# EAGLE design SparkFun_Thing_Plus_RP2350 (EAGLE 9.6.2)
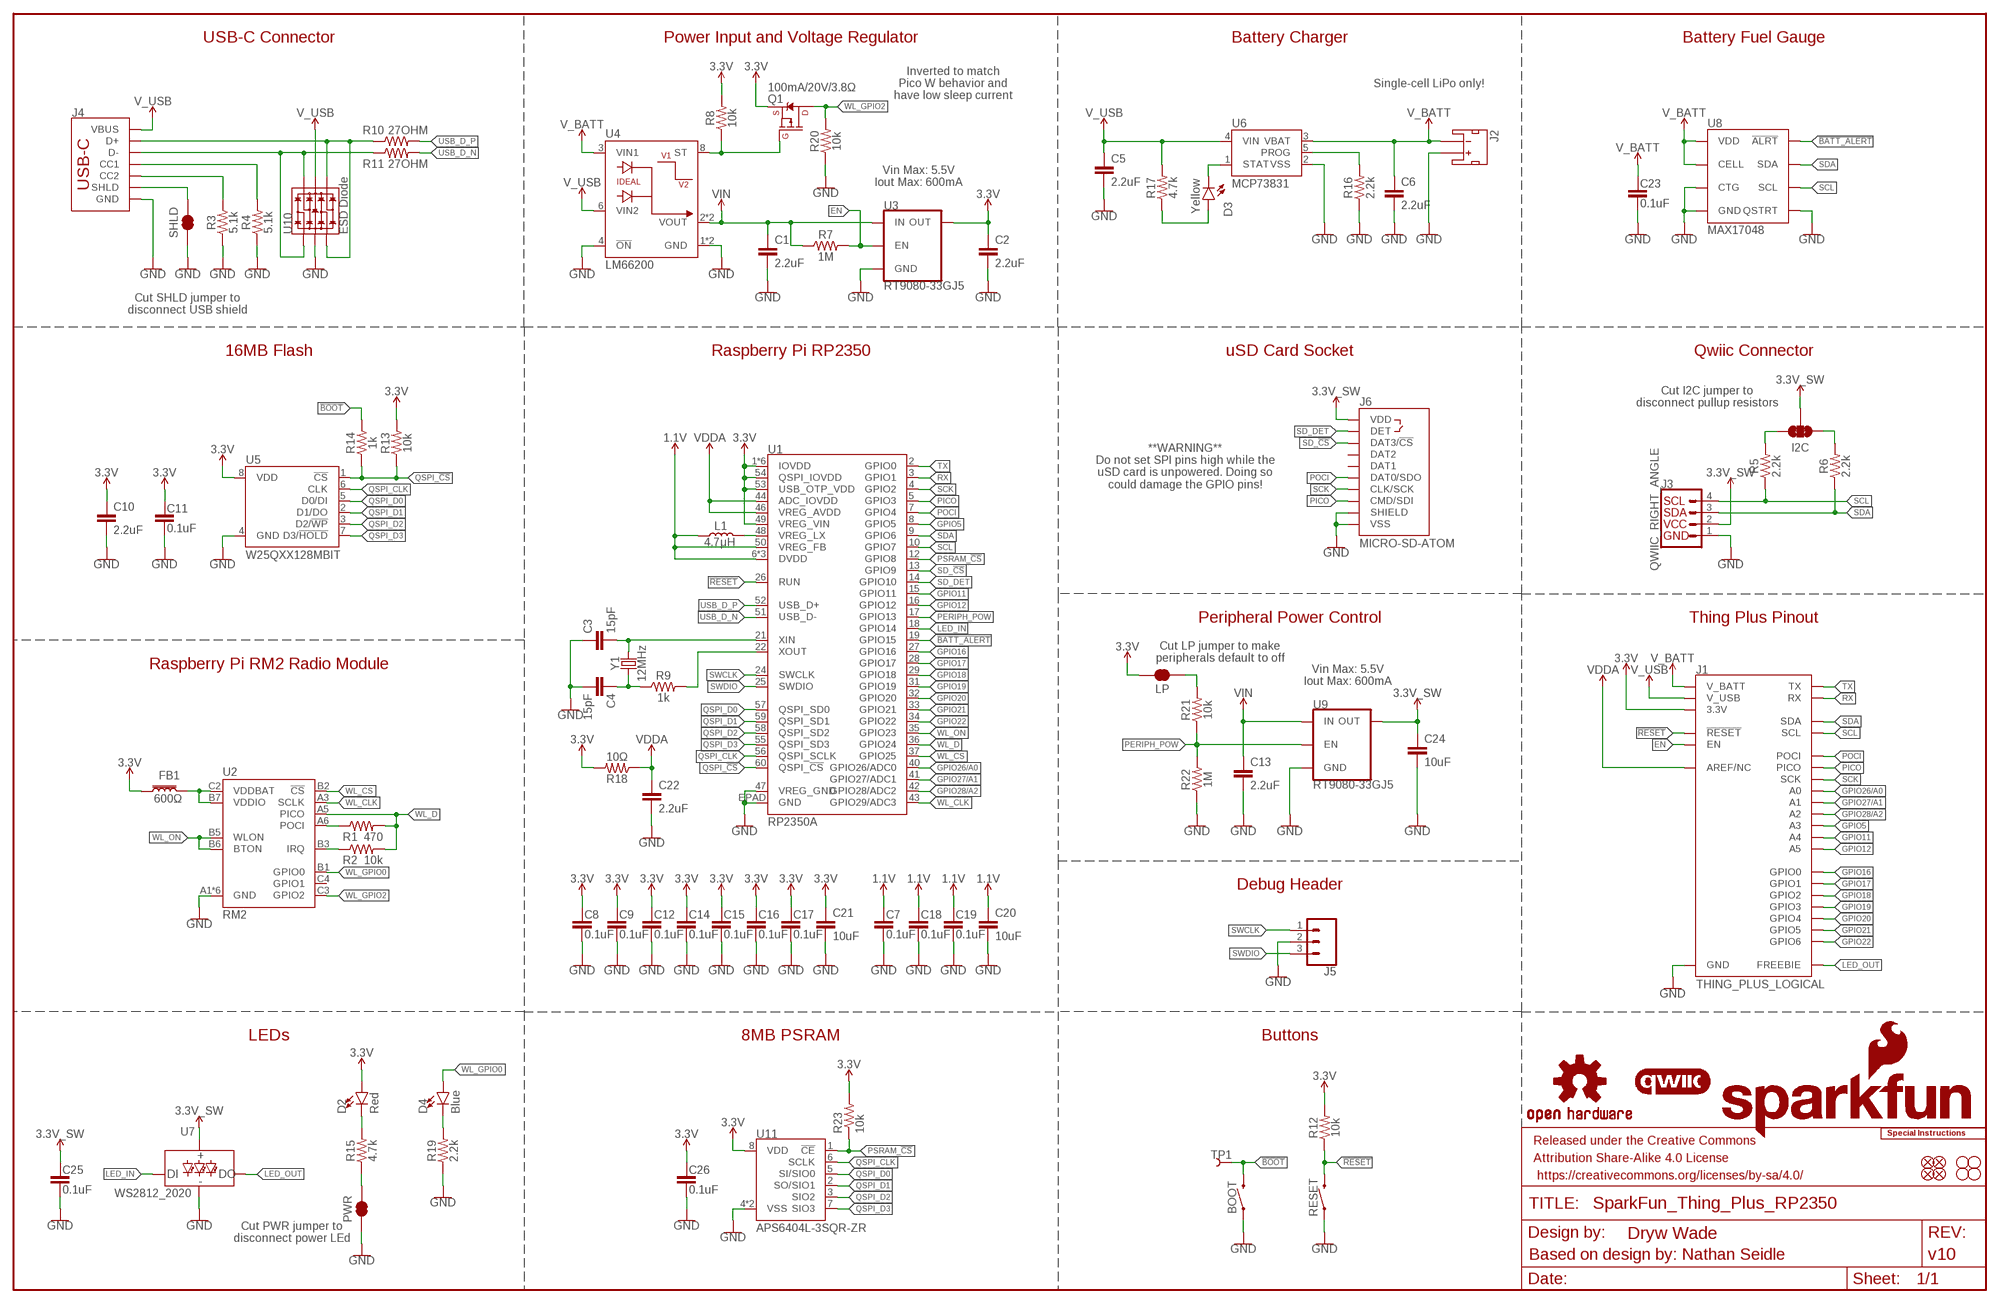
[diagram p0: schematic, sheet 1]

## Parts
BOOT  MOMENTARY-SWITCH-SPST-SMD-4.6X2.8MM  [TACTILE_SWITCH_SMD_4.6X2.8MM]
C1  2.2uF  2.2UF-0402_TIGHT-10V-10%-X5R  [0402-TIGHT]
C2  2.2uF  2.2UF-0402_TIGHT-10V-10%-X5R  [0402-TIGHT]
C3  15pF  15PF-0402T-50V-5%  [0402-TIGHT]
C4  15pF  15PF-0402T-50V-5%  [0402-TIGHT]
C5  2.2uF  2.2UF-0402_TIGHT-10V-10%-X5R  [0402-TIGHT]
C6  2.2uF  2.2UF-0402_TIGHT-10V-10%-X5R  [0402-TIGHT]
C7  0.1uF  0.1UF-0402T-6.3V-10%-X7R  [0402-TIGHT]
C8  0.1uF  0.1UF-0402T-6.3V-10%-X7R  [0402-TIGHT]
C9  0.1uF  0.1UF-0402T-6.3V-10%-X7R  [0402-TIGHT]
C10  2.2uF  2.2UF-0402_TIGHT-10V-10%-X5R  [0402-TIGHT]
C11  0.1uF  0.1UF-0402T-6.3V-10%-X7R  [0402-TIGHT]
C12  0.1uF  0.1UF-0402T-6.3V-10%-X7R  [0402-TIGHT]
C13  2.2uF  2.2UF-0402_TIGHT-10V-10%-X5R  [0402-TIGHT]
C14  0.1uF  0.1UF-0402T-6.3V-10%-X7R  [0402-TIGHT]
C15  0.1uF  0.1UF-0402T-6.3V-10%-X7R  [0402-TIGHT]
C16  0.1uF  0.1UF-0402T-6.3V-10%-X7R  [0402-TIGHT]
C17  0.1uF  0.1UF-0402T-6.3V-10%-X7R  [0402-TIGHT]
C18  0.1uF  0.1UF-0402T-6.3V-10%-X7R  [0402-TIGHT]
C19  0.1uF  0.1UF-0402T-6.3V-10%-X7R  [0402-TIGHT]
C20  10uF  10UF-0402T-6.3V-20%  [0402-TIGHT]
C21  10uF  10UF-0402T-6.3V-20%  [0402-TIGHT]
C22  2.2uF  2.2UF-0402_TIGHT-10V-10%-X5R  [0402-TIGHT]
C23  0.1uF  0.1UF-0402T-6.3V-10%-X7R  [0402-TIGHT]
C24  10uF  10UF-0402T-6.3V-20%  [0402-TIGHT]
C25  0.1uF  0.1UF-0402T-6.3V-10%-X7R  [0402-TIGHT]
C26  0.1uF  0.1UF-0402T-6.3V-10%-X7R  [0402-TIGHT]
D2  Red  LED-RED_0603-KB  [LED-0603]
D3  Yellow  LED-YELLOW0603  [LED-0603]
D4  Blue  LED-BLUE0603  [LED-0603]
FB1  600Ω  FERRITE_BEAD-0805-600Ω-100MHZ  [0805]
FD1  FIDUCIALUFIDUCIAL  [FIDUCIAL-MICRO]
FD2  FIDUCIALUFIDUCIAL  [FIDUCIAL-MICRO]
FD3  FIDUCIALUFIDUCIAL  [FIDUCIAL-MICRO]
FD4  FIDUCIALUFIDUCIAL  [FIDUCIAL-MICRO]
FRAME1  FRAME-LEDGER  [CREATIVE_COMMONS]
H1  STAND-OFF  [STAND-OFF]
H2  STAND-OFF  [STAND-OFF]
H3  STAND-OFF  [STAND-OFF]
H4  STAND-OFF  [STAND-OFF]
I2C  JUMPER-SMT_3_2-NC_TRACE_SILK  [SMT-JUMPER_3_2-NC_TRACE_SILK]
J1  THING_PLUS_LOGICAL  [THING_PLUS]
J2  JST_2MM_MALE  [JST-2-SMD]
J3  QWIIC_RIGHT_ANGLE  QWIIC_CONNECTORJS-1MM  [JST04_1MM_RA]
J4  USB_C_4-LAYER_PADS  [USB-C-16P_4LAYER-PADS]
J5  CONN_031X03_NO_SILK  [1X03_NO_SILK]
J6  MICRO-SD-ATOM  [MICROSD_ATOM]
L1  4.7μH  4.7μH_SHIELDED_INDUCTOR  [1008(2520)]
LOGO1  SFE_LOGO_NAME_FLAME.1_INCH  [SFE_LOGO_NAME_FLAME_.1]
LOGO2  OSHW-LOGOS  [OSHW-LOGO-S]
LOGO3  QWIIC_LOGO_4MM  [QWIIC_4MM]
LOGO5  SPECIAL_INSTRUCTIONS-ORDERING  [ORDERING_INSTRUCTIONS]
LP  JUMPER-SMT_2_NC_TRACE_SILK  [SMT-JUMPER_2_NC_TRACE_SILK]
PWR  JUMPER-SMT_2_NC_TRACE_SILK  [SMT-JUMPER_2_NC_TRACE_SILK]
Q1  100mA/20V/3.8Ω  MOSFET_PCH-RE1C001ZPTL  [SOT-416FL]
R1  470  470OHM-0402-TIGHT-1/16W-1%  [0402-TIGHT]
R2  10k  10KOHM-0402T-1/16W-1%  [0402-TIGHT]
R3  5.1k  5.1KOHM-0402T-1/16W-1%  [0402-TIGHT]
R4  5.1k  5.1KOHM-0402T-1/16W-1%  [0402-TIGHT]
R5  2.2k  2.2KOHM-0402T-1/16W-1%  [0402-TIGHT]
R6  2.2k  2.2KOHM-0402T-1/16W-1%  [0402-TIGHT]
R7  1M  1MOHM-0402T-1/16W-5%  [0402-TIGHT]
R8  10k  10KOHM-0402T-1/16W-1%  [0402-TIGHT]
R9  1k  1KOHM-0402T-1/16W-1%  [0402-TIGHT]
R10  27OHM  [0402-TIGHT]
R11  27OHM  [0402-TIGHT]
R12  10k  10KOHM-0402T-1/16W-1%  [0402-TIGHT]
R13  10k  10KOHM-0402T-1/16W-1%  [0402-TIGHT]
R14  1k  1KOHM-0402T-1/16W-1%  [0402-TIGHT]
R15  4.7k  4.7KOHM-0402T-1/16W-1%  [0402-TIGHT]
R16  2.2k  2.2KOHM-0402T-1/16W-1%  [0402-TIGHT]
R17  4.7k  4.7KOHM-0402T-1/16W-1%  [0402-TIGHT]
R18  10Ω  10OHM-0402-1/16W-5%  [0402-TIGHT]
R19  2.2k  2.2KOHM-0402T-1/16W-1%  [0402-TIGHT]
R20  10k  10KOHM-0402T-1/16W-1%  [0402-TIGHT]
R21  10k  10KOHM-0402T-1/16W-1%  [0402-TIGHT]
R22  1M  1MOHM-0402T-1/16W-5%  [0402-TIGHT]
R23  10k  10KOHM-0402T-1/16W-1%  [0402-TIGHT]
RESET  MOMENTARY-SWITCH-SPST-SMD-4.6X2.8MM  [TACTILE_SWITCH_SMD_4.6X2.8MM]
SHLD  JUMPER-SMT_2_NC_TRACE_SILK  [SMT-JUMPER_2_NC_TRACE_SILK]
TP1  TEST-POINT3X5  [PAD.03X.05]
U1  RP2350A  [RP2350A]
U2  RM2  [RM2]
U3  RT9080-33GJ5  V_REG_RT9080-33GJ5  [SOT23-5]
U4  LM66200  IDEAL_DIODE_DUAL_LM66200  [SOT8]
U5  W25QXX128MBIT  W25QXX128MBIT-6X5-SKINNY_CENTER  [WSON-8-6X5-SKINNY_CENTERPAD]
U6  MCP73831  [SOT23-5]
U7  WS2812_2020  [WS2812-2020]
U8  MAX17048  MAX17048DFN8  [DFN-8]
U9  RT9080-33GJ5  V_REG_RT9080-33GJ5  [SOT23-5]
U10  ESD Diode  TVS_DIODE_ARRAY_DT1042-04SO-7  [SOT-23-6]
U11  APS6404L-3SQR-ZR  [APS6404L-3SQR-ZR]
Y1  12MHz  CRYSTAL-12MHZ  [CRYSTAL-SMD-2X2.5MM]

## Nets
1.1V: C7.1 C18.1 C19.1 C20.1 L1.1 U1.6(DVDD) U1.23(DVDD) U1.39(DVDD) U1.50(VREG_FB)
3.3V: C2.1 C8.1 C9.1 C10.1 C11.1 C12.1 C14.1 C15.1 C16.1 C17.1 C21.1 C26.1 D2.A FB1.1 J1.27(3.3V) LP.2 Q1.2(S) R8.2 R12.2 R13.2 R18.2 R23.2 U1.1(IOVDD) U1.11(IOVDD) U1.20(IOVDD) U1.30(IOVDD) U1.38(IOVDD) U1.45(IOVDD) U1.49(VREG_VIN) U1.53(USB_OTP_VDD) U1.54(QSPI_IOVDD) U3.5(OUT) U5.8(VDD) U11.8(VDD)
3.3V_SW: C24.1 C25.1 I2C.2 J3.2 J6.4(VDD) U7.VCC U9.5(OUT)
!BATT_ALERT!: U1.19(GPIO15) U8.5(!ALRT)
!BOOT!: BOOT.3 BOOT.4 R14.2 TP1.1
!RESET!: J1.28(!RESET) R12.1 RESET.3 RESET.4 U1.26(RUN)
BAT_SW: Q1.1(G) R8.1 U4.8(ST)
EN: J1.11(EN) R7.2 U3.3(EN)
GND: BOOT.1 BOOT.2 C1.2 C2.2 C3.1 C4.2 C5.2 C6.2 C7.2 C8.2 C9.2 C10.2 C11.2 C12.2 C13.2 C14.2 C15.2 C16.2 C17.2 C18.2 C19.2 C20.2 C21.2 C22.2 C23.2 C24.2 C25.2 C26.2 J1.25(GND) J2.2(+) J3.1 J4.GND J4.GND2(GND) J5.2 J6.6(VSS) J6.SHIELD1(SHIELD) J6.SHIELD2(SHIELD) J6.SHIELD3(SHIELD) J6.SHIELD4(SHIELD) PWR.1 R3.1 R4.1 R16.1 R19.1 R20.1 R22.1 RESET.1 RESET.2 SHLD.1 U1.47(VREG_GND) U1.EPAD(GND) U2.A1(GND) U2.A4(GND) U2.A7(GND) U2.B4(GND) U2.C1(GND) U2.C7(GND) U3.2(GND) U4.1(GND) U4.4(!ON!) U4.5(GND) U5.4(GND) U6.2(VSS) U7.GND U8.1(CTG) U8.4(GND) U8.6(QSTRT) U8.9(GND) U9.2(GND) U10.2(VSS) U11.4(VSS) U11.9(VSS)
GPIO5: J1.21(A3) U1.8(GPIO5)
GPIO11: J1.20(A4) U1.15(GPIO11)
GPIO12: J1.19(A5) U1.16(GPIO12)
GPIO16: J1.9(GPIO0) U1.27(GPIO16)
GPIO17: J1.8(GPIO1) U1.28(GPIO17)
GPIO18: J1.7(GPIO2) U1.29(GPIO18)
GPIO19: J1.6(GPIO3) U1.31(GPIO19)
GPIO20: J1.5(GPIO4) U1.32(GPIO20)
GPIO21: J1.4(GPIO5) U1.33(GPIO21)
GPIO22: J1.3(GPIO6) U1.34(GPIO22)
GPIO26/A0: J1.24(A0) U1.40(GPIO26/ADC0)
GPIO27/A1: J1.23(A1) U1.41(GPIO27/ADC1)
GPIO28/A2: J1.22(A2) U1.42(GPIO28/ADC2)
LED_IN: U1.18(GPIO14) U7.DI
LED_OUT: J1.13(FREEBIE) U7.DO
N$1: FB1.2 U2.B7(VDDIO) U2.C2(VDDBAT)
N$2: R1.1 U2.A6(POCI)
N$3: R2.1 U2.B3(IRQ)
N$4: D4.C R19.2
N$5: J4.B5(CC2) R3.2
N$6: J4.A5(CC1) R4.2
N$7: J4.A7(D-) J4.B7(D-) R11.1 U10.1(IO1) U10.6(IO4)
N$8: J4.A6(D+) J4.B6(D+) R10.1 U10.3(IO2) U10.4(IO3)
N$9: I2C.3 R5.2
N$10: I2C.1 R6.2
N$11: LP.1 R21.2
N$13: C3.2 U1.21(XIN) Y1.P3
N$14: C4.1 R9.1 Y1.P1
N$15: R9.2 U1.22(XOUT)
N$18: D2.C R15.2
N$19: PWR.2 R15.1
N$20: R16.2 U6.5(PROG)
N$21: D3.A R17.1
N$22: D3.C U6.1(STAT)
N$23: L1.2 U1.48(VREG_LX)
PERIPH_POW: R21.1 R22.2 U1.17(GPIO13) U9.3(EN)
PICO: J1.17(PICO) J6.3(CMD/SDI) U1.5(GPIO3)
POCI: J1.16(POCI) J6.7(DAT0/SDO) U1.7(GPIO4)
PSRAM_!CS!: R23.1 U1.12(GPIO8) U11.1(!CE!)
QSPI_!CS!: R13.1 R14.1 U1.60(QSPI_!CS!) U5.1(!CS!)
QSPI_CLK: U1.56(QSPI_SCLK) U5.6(CLK) U11.6(SCLK)
QSPI_D0: U1.57(QSPI_SD0) U5.5(D0/DI) U11.5(SI/SIO0)
QSPI_D1: U1.59(QSPI_SD1) U5.2(D1/DO) U11.2(SO/SIO1)
QSPI_D2: U1.58(QSPI_SD2) U5.3(D2/!WP!) U11.3(SIO2)
QSPI_D3: U1.55(QSPI_SD3) U5.7(D3/!HOLD!) U11.7(SIO3)
RX: J1.15(RX) U1.3(GPIO1)
SCK: J1.18(SCK) J6.5(CLK/SCK) U1.4(GPIO2)
SCL: J1.2(SCL) J3.4 R5.1 U1.10(GPIO7) U8.7(SCL)
SD_!CS!: J6.2(DAT3/!CS!) U1.13(GPIO9)
SD_DET: J6.9(DET) U1.14(GPIO10)
SDA: J1.1(SDA) J3.3 R6.1 U1.9(GPIO6) U8.8(SDA)
SHLD: J4.SHLD1(SHLD) J4.SHLD2(SHLD) J4.SHLD3(SHLD) J4.SHLD4(SHLD) SHLD.2
SWCLK: J5.1 U1.24(SWCLK)
SWDIO: J5.3 U1.25(SWDIO)
TX: J1.14(TX) U1.2(GPIO0)
USB_D_N [USB]: R11.2 U1.51(USB_D-)
USB_D_P [USB]: R10.2 U1.52(USB_D+)
V_BATT: C6.1 C23.1 J1.12(V_BATT) J2.1(-) U4.3(VIN1) U6.3(VBAT) U8.2(CELL) U8.3(VDD)
V_USB: C5.1 J1.10(V_USB) J4.VBUS1(VBUS) J4.VBUS2(VBUS) R17.2 U4.6(VIN2) U6.4(VIN) U10.5(VCC)
VDDA: C22.1 J1.26(AREF/NC) R18.1 U1.44(ADC_IOVDD) U1.46(VREG_AVDD)
VIN: C1.1 C13.1 R7.1 U3.1(IN) U4.2(VOUT) U4.7(VOUT) U9.1(IN)
WL_CLK: U1.43(GPIO29/ADC3) U2.A3(SCLK)
WL_CS: U1.37(GPIO25) U2.B2(!CS!)
WL_D: R1.2 R2.2 U1.36(GPIO24) U2.A5(PICO)
WL_GPIO0: D4.A U2.B1(GPIO0)
WL_GPIO2: Q1.3(D) R20.2 U2.C3(GPIO2)
WL_ON: U1.35(GPIO23) U2.B5(WLON) U2.B6(BTON)
Unconnected: J2.NC1(PAD1) J2.NC2(PAD2) J6.1(DAT2) J6.8(DAT1) U2.C4(GPIO1)

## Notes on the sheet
- USB-C Connector | Power Input and Voltage Regulator | Battery Charger | Battery Fuel Gauge
- Inverted to match
  Pico W behavior and
  have low sleep current
- Single-cell LiPo only!
- Vin Max: 5.5V
  Iout Max: 600mA
- Cut SHLD jumper to
  disconnect USB shield
- 16MB Flash | Raspberry Pi RP2350 | uSD Card Socket | Qwiic Connector
- Cut I2C jumper to
  disconnect pullup resistors
- **WARNING**
  Do not set SPI pins high while the
  uSD card is unpowered. Doing so
  could damage the GPIO pins!
- Peripheral Power Control | Thing Plus Pinout
- Cut LP jumper to make
  peripherals default to off
- Raspberry Pi RM2 Radio Module
- Vin Max: 5.5V
  Iout Max: 600mA
- Debug Header
- LEDs | 8MB PSRAM | Buttons
- Cut PWR jumper to
  disconnect power LEd
- Based on design by: Nathan Seidle

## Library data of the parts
BOOT RESET = SparkFun-Switches:MOMENTARY-SWITCH-SPST: Momentary Switch (Pushbutton) - SPST; PROD_ID: SWCH-15606
C1 C2 C5 C6 C10 C13 C22 = SparkFun-Capacitors:2.2UF: 2.2µF ceramic capacitors; PROD_ID: CAP-14232
C3 C4 = SparkFun-Capacitors:15PF: 15pF ceramic capacitors; PROD_ID: CAP-13063
C7-C9 C11 C12 C14-C19 C23 C25 C26 = SparkFun-Capacitors:0.1UF: 0.1µF ceramic capacitors; PROD_ID: CAP-14993
C20 C21 C24 = SparkFun-Capacitors:10UF: 10.0µF ceramic capacitors; PROD_ID: CAP-14848
D2 = SparkFun-LED:LED-RED: Red SMD LED; PROD_ID: DIO-17976
D3 = SparkFun-LED:LED-YELLOW: Yellow SMD LED; PROD_ID: DIO-09003
D4 = SparkFun-LED:LED-BLUE: Blue SMD LED; PROD_ID: DIO-08575
FB1 = SparkFun-Coils:FERRITE_BEAD: Ferrite Bead (blocks, cores, rings, chokes, etc.); PROD_ID: NDUC-14988
FD1-FD4 = SparkFun-Aesthetics:FIDUCIAL: Fiducial Alignment Points
FRAME1 = SparkFun-Aesthetics:FRAME-LEDGER: Schematic Frame - Ledger; DESIGNER: Dryw Wade; REV: v10
H1-H4 = SparkFun-Hardware:STAND-OFF: Stand Off
I2C = SparkFun-Jumpers:JUMPER-SMT_3_2-NC_TRACE: Normally closed trace jumper (2 of 2 connections) This jumper has a trace between all three pads so they are normally closed (NC). Use a razor knife to open the connection(s). For best results follow the IPC guidelines for cutting traces: Cutout at least 0.063 mm (0.005 in). Remove all loose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
J1 = SparkFun-Boards:THING_PLUS_LOGICAL
J2 = SparkFun-Connectors:JST_2MM_MALE: JST 2MM MALE RA CONNECTOR Two pin, compact surface mount connector. Commonly used as a battery input connection point. We really like the solid locking feeling and high current rating on these small connectors. We use these all the time as battery connectors. Mates to single-cell LiPo batteries.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; PROD_ID: CONN-11443; SF_ID: PRT-08612
J3 = SparkFun-Connectors:QWIIC_CONNECTOR: SparkFun I2C Standard Qwiic Connector An SMD 1mm pitch JST connector makes it easy and quick (get it? Qwiic?) to connect I2C devices to each other. The Qwiic system enables fast and solderless connection between popular platforms and various sensors and actuators. We carry 200mm, 100mm, 50mm, and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; PROD_ID: CONN-13694
J4 = SparkFun-Connectors:USB_C: USB Type C 16Pin Connector Super Speed pins not available on the 16-pin purely SMD connector so this part is best for USB 2.0 implementations. D1 and D2 are tied together enabling D+/- no matter which way the cable is plugged into the connector. The two channel configuration pins (CC1/2) are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; PROD_ID: CONN-14122
J5 = SparkFun-Connectors:CONN_03: Multi connection point. Often used as Generic Header-pin footprint for 0.1 inch spaced/style header connections On any of the 0.1 inch spaced packages, you can populate with these: Break Away Headers - Straight (PRT-00116) Break Away Male Headers - Right Angle (PRT-00553) Female Headers (PRT-00115)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
J6 = SparkFun-Connectors:MICRO-SD-ATOM; PROD_ID: CONN-20948
L1 = SparkFun-Coils:4.7μH_SHIELDED_INDUCTOR: 4.7uH Inductor; PROD_ID: NDUC-14880
LOGO1 = SparkFun-Aesthetics:SFE_LOGO_NAME_FLAME: SparkFun Font Logo w/ Flame
LOGO2 = SparkFun-Aesthetics:OSHW-LOGO: Open-Source Hardware (OSHW) Logo
LOGO3 = SparkFun-Aesthetics:QWIIC_LOGO: Qwiic Logos for placement on schematic and PCB. The 5.5mm silk logo is best for placing next to Qwiic connector.
LOGO5 = SparkFun-Aesthetics:SPECIAL_INSTRUCTIONS: Special Ordering/Production Instructions Alert
LP PWR SHLD = SparkFun-Jumpers:JUMPER-SMT_2_NC_TRACE: Normally closed trace jumper
Q1 = SparkFun-DiscreteSemi:MOSFET_PCH: P-channel MOSFETs Voltage controlled devices that allow control of high current outputs. SparkFun Products: SparkFun ESP32 Thing SparkFun ESP8266 Thing SparkFun Pi Servo HAT V2 DMG2305UX-7 (20V/4.2A/SOT23-3); PROD_ID: TRANS-15421
R1 = SparkFun-Resistors:470OHM: 470Ω resistor; PROD_ID: RES-15584
R2 R8 R12 R13 R20 R21 R23 = SparkFun-Resistors:10KOHM: 10kΩ resistor; PROD_ID: RES-14241
R3 R4 = SparkFun-Resistors:5.1KOHM; PROD_ID: RES-14340
R5 R6 R16 R19 = SparkFun-Resistors:2.2KOHM: 2.2kΩ resistor; PROD_ID: RES-14341
R7 R22 = SparkFun-Resistors:1MOHM: 1MΩ resistor; PROD_ID: RES-15185
R9 R14 = SparkFun-Resistors:1KOHM: 1kΩ resistor; PROD_ID: RES-14342
R10 R11 = SparkFun-Resistors:27OHM: 27Ω resistor; PROD_ID: RES-15238
R15 R17 = SparkFun-Resistors:4.7KOHM: 4.7kΩ resistor; PROD_ID: RES-15343
R18 = SparkFun-Resistors:10OHM: 10Ω resistor; PROD_ID: RES-16072
TP1 = SparkFun-Connectors:TEST-POINT: SparkFun Test Points
U1 = RP2350A:RP2350A; PROD_ID: IC-21276
U2 = RM2:RM2; PROD_ID: IC-21607
U3 U9 = SparkFun-IC-Power:V_REG_RT9080-33GJ5: RT9080-33GJ5 Low-Dropout Linear Regulator The RT9080 is a low-dropout (LDO) voltage regulators with enable function that operates from 1.2V to 5.5V. It provides up to 600mA of output current and offers low-power operation in miniaturized packaging. The features of low quiescent current as low as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; PROD_ID: VREG-19034
U4 = SparkFun-IC-Power:IDEAL_DIODE_DUAL_LM66200; PROD_ID: IC-20783
U5 = SparkFun-IC-Memory:W25QXX; PROD_ID: IC-15107
U6 = SparkFun-IC-Power:MCP73831: MCP73831T Li-Ion, Li-Pol Controller Miniature single cell, fully integrated Li-Ion, Li-polymer charge management controller Datasheet SparkFun Products: SparkFun ESP32 Thing SparkFun 9DoF Razor IMU M0; PROD_ID: IC-09995
U7 = SparkFun-LED:WS2812: Addressable RGB LED - 1 Wire Common names: WS2812, SK6812, Neopixel, APA-106, etc. SMD LED with built-in controller IC. Color: Red/Green/Blue SparkFun Products: LED-SMD RGB (WS2812) LED - RGB Addressable, PTH, 5mm Diffused (5 Pack) LED - RGB Addressable, PTH, 5mm Clear (5 Pack) RGB Addressable CBI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; PROD_ID: DIO-15591
U8 = SparkFun-IC-Power:MAX17048: Micropower 1-Cell Li+ ModelGauge SparkFun Products Qduino Mini (DEV-13614); PROD_ID: IC-12551
U10 = SparkFun-DiscreteSemi:TVS_DIODE_ARRAY; PROD_ID: IC-13538
U11 = RP2350A:APS6404L-3SQR-ZR; PROD_ID: IC-21870
Y1 = SparkFun-Clocks:CRYSTAL-12MHZ: 12.0MHz Crystal; PROD_ID: XTAL-15540

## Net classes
1 USB: width 0.233 mm, clearance 0.127 mm to class 0, clearance 0.127 mm

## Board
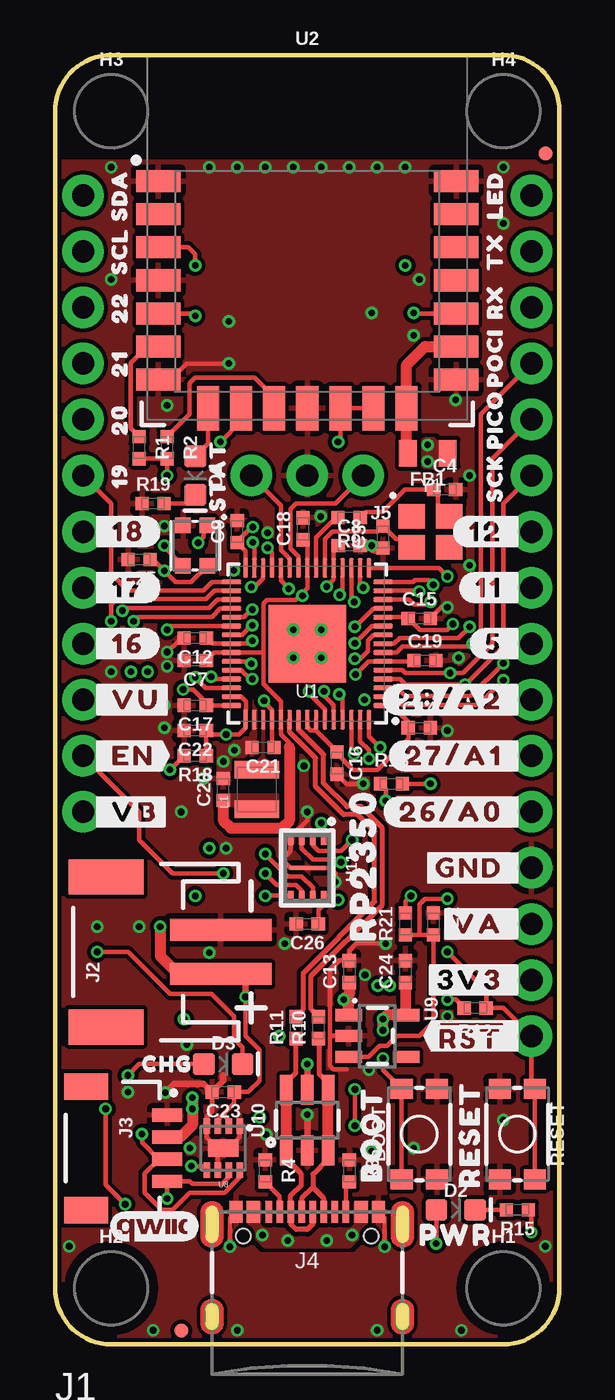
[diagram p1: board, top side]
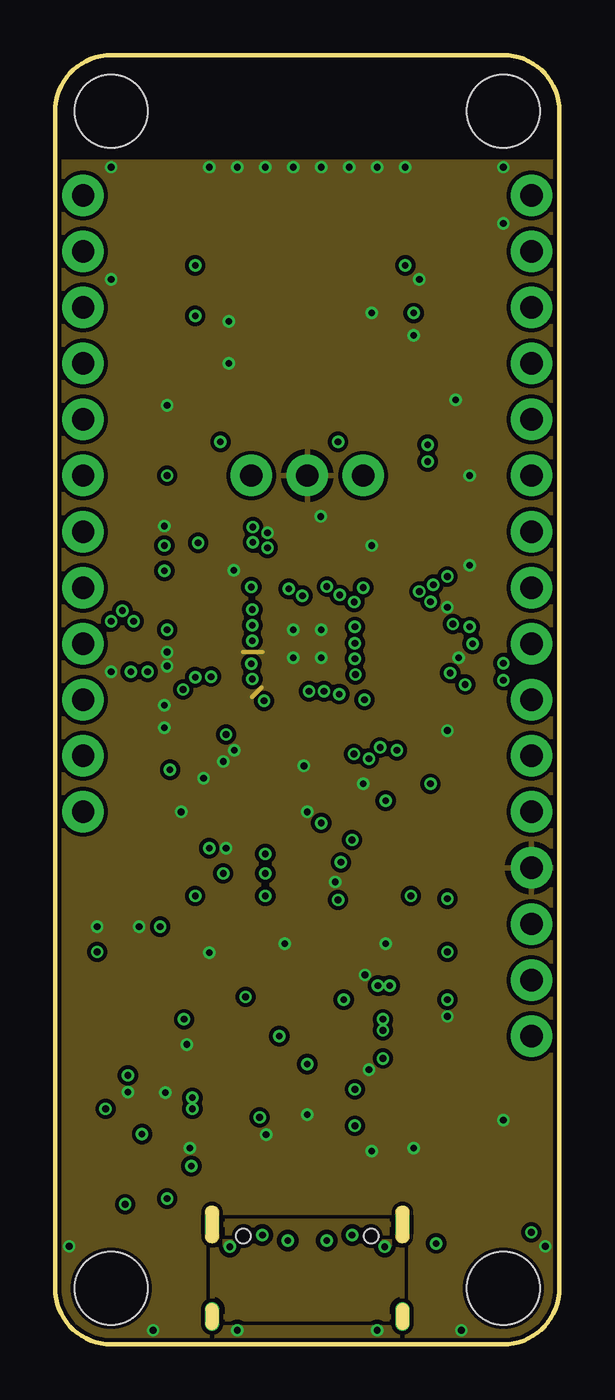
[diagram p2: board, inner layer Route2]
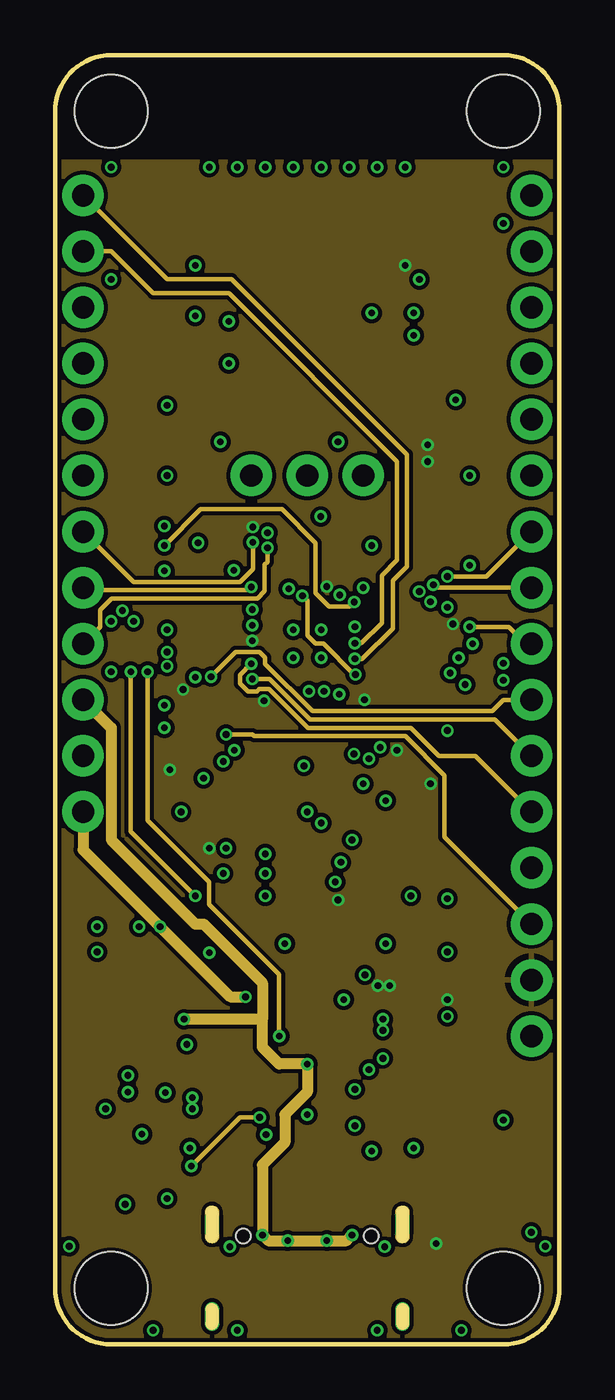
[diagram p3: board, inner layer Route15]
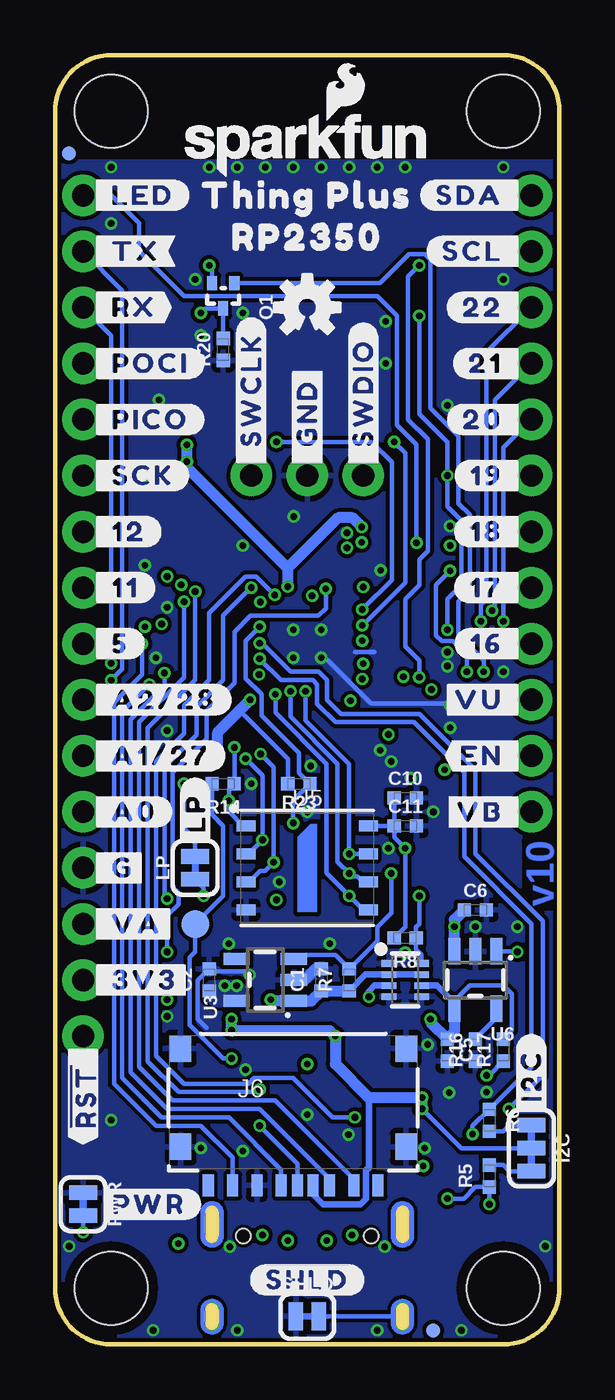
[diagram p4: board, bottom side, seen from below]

Size 22.86 x 58.42 mm. Coordinates in mm from the lower left corner, seen from the top.
Outline: 2.54,0 20.32,0 arc90 22.86,2.54 22.86,55.88 arc90 20.32,58.42 2.54,58.42 arc90 0,55.88 0,2.54 arc90 2.54,0
Copper layers (1*2*15*16): Top 0.035559375mm / dielectric 0.47751875mm / Route2 0.035559375mm / dielectric 0.47751875mm / Route15 0.035559375mm / dielectric 0.47751875mm / Bottom 0.035559375mm
Design rules "SparkFun-4-Layer-Minimum-JLCPCB": minimum track width 5mil, minimum drill 0.2mm, track to track 5mil, track to pad 5mil, pad to pad 5mil, via to via 5mil, smd to smd 5mil, copper to edge 7mil, drill to drill 7mil, minimum pad ring 5mil, minimum via ring 5mil, stop-mask expansion 2.5mil, vias tented up to drill 25mil, thermal gap 10mil

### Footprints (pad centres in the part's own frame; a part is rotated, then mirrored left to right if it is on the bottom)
TACTILE_SWITCH_SMD_4.6X2.8MM = smd 0.9 x 1: 1 -2.05,-0.8; 2 2.05,-0.8; 3 2.05,0.8; 4 -2.05,0.8
0402-TIGHT = smd 0.6 x 0.6: 1 -0.5,0; 2 0.5,0
LED-0603 = smd 1 x 1: A -0.877,0; C 0.877,0
0805 = smd 0.8 x 1.2: 1 -0.9,0; 2 0.9,0
FIDUCIAL-MICRO = smd 0.635 x 0.635: 1 0,0
STAND-OFF = hole 3.302: 0,0
SMT-JUMPER_3_2-NC_TRACE_SILK = smd 0.66 x 1.27: 1 -1.041,0; 2 0,0; 3 1.041,0
THING_PLUS = drill 1.016 pad 1.88: 1 1.27,52.07; 2 1.27,49.53; 3 1.27,46.99; 4 1.27,44.45; 5 1.27,41.91; 6 1.27,39.37; 7 1.27,36.83; 8 1.27,34.29; 9 1.27,31.75; 10 1.27,29.21; 11 1.27,26.67; 12 1.27,24.13; 13 21.59,52.07; 14 21.59,49.53; 15 21.59,46.99; 16 21.59,44.45; 17 21.59,41.91; 18 21.59,39.37; 19 21.59,36.83; 20 21.59,34.29; 21 21.59,31.75; 22 21.59,29.21; 23 21.59,26.67; 24 21.59,24.13; 25 21.59,21.59; 26 21.59,19.05; 27 21.59,16.51; 28 21.59,13.97
JST-2-SMD = smd 1 x 4.6: 1 -1,-3.7; 2 1,-3.7 | smd 1.6 x 3.4: NC1 -3.4,1.5; NC2 3.4,1.5
JST04_1MM_RA = smd 0.6 x 1.35: 1 -1.5,0; 2 -0.5,0; 3 0.5,0; 4 1.5,0 | smd 1.2 x 2: NC1 2.8,-3.675; NC2 -2.8,-3.675
USB-C-16P_4LAYER-PADS = smd 0.3 x 1: A5 -1.25,-0.34; A6 -0.25,-0.34; A7 0.25,-0.34; A8 1.25,-0.34; B5 1.75,-0.34; B6 0.75,-0.34; B7 -0.75,-0.34; B8 -1.75,-0.34 | smd 0.6 x 1: GND -3.225,-0.34; GND2 3.225,-0.34; VBUS1 -2.45,-0.34; VBUS2 2.45,-0.34 | drill 0.4 pad 0.6 long: SHLD1 -4.318,-0.915; SHLD2 4.318,-0.915; SHLD3 -4.318,-5.095; SHLD4 4.318,-5.095 | hole 0.65: -2.89,-1.445; 2.89,-1.445
1X03_NO_SILK = drill 1.016 pad 1.88: 1 0,0; 2 2.54,0; 3 5.08,0
MICROSD_ATOM = smd 0.5 x 1: 1 3.85,-3.975; 2 2.75,-3.975; 3 1.65,-3.975; 4 0.9,-3.975; 5 -0.55,-3.975; 6 -1.65,-3.975; 7 -2.75,-3.975; 8 -3.85,-3.975; 9 0.2,-3.975 | smd 0.95 x 1.2: SHIELD1 5.1,-2.225; SHIELD2 5.1,2.225; SHIELD3 -5.1,2.225; SHIELD4 -5.1,-2.225
1008(2520) = smd 0.8 x 2: 1 -0.9,0; 2 0.9,0
SMT-JUMPER_2_NC_TRACE_SILK = smd 0.66 x 1.27: 1 -0.521,0; 2 0.521,0
SOT-416FL = smd 0.46 x 0.65: 1 -0.5,-1.1; 2 0.5,-1.1; 3 0,0.05
PAD.03X.05 = smd 1.27 x 1.27: 1 0,0
RP2350A = smd 0.875 x 0.2: 1 -3.437,2.8; 2 -3.437,2.4; 3 -3.437,2; 4 -3.437,1.6; 5 -3.437,1.2; 6 -3.437,0.8; 7 -3.437,0.4; 8 -3.437,0; 9 -3.437,-0.4; 10 -3.437,-0.8; 11 -3.437,-1.2; 12 -3.437,-1.6; 13 -3.437,-2; 14 -3.437,-2.4; 15 -3.437,-2.8; 31 3.437,-2.8; 32 3.437,-2.4; 33 3.437,-2; 34 3.437,-1.6; 35 3.437,-1.2; 36 3.437,-0.8; 37 3.437,-0.4; 38 3.437,0; 39 3.437,0.4; 40 3.437,0.8; 41 3.437,1.2; 42 3.437,1.6; 43 3.437,2; 44 3.437,2.4; 45 3.437,2.8 | smd 0.2 x 0.875: 16 -2.8,-3.437; 17 -2.4,-3.437; 18 -2,-3.437; 19 -1.6,-3.437; 20 -1.2,-3.437; 21 -0.8,-3.437; 22 -0.4,-3.437; 23 0,-3.437; 24 0.4,-3.437; 25 0.8,-3.437; 26 1.2,-3.437; 27 1.6,-3.437; 28 2,-3.437; 29 2.4,-3.437; 30 2.8,-3.437; 46 2.8,3.437; 47 2.4,3.437; 48 2,3.437; 49 1.6,3.437; 50 1.2,3.437; 51 0.8,3.437; 52 0.4,3.437; 53 0,3.437; 54 -0.4,3.437; 55 -0.8,3.437; 56 -1.2,3.437; 57 -1.6,3.437; 58 -2,3.437; 59 -2.4,3.437; 60 -2.8,3.437 | smd 3.5 x 3.5: EPAD 0,0
RM2 = smd 2 x 1: A1 -6.75,2.55; A2 -6.75,1.05; A3 -6.75,-0.45; A4 -6.75,-1.95; A5 -6.75,-3.45; A6 -6.75,-4.95; A7 -6.75,-6.45; C1 6.75,-6.45; C2 6.75,-4.95; C3 6.75,-3.45; C4 6.75,-1.95; C5 6.75,-0.45; C6 6.75,1.05; C7 6.75,2.55 | smd 1 x 2: B1 -4.5,-7.75; B2 -3,-7.75; B3 -1.5,-7.75; B4 0,-7.75; B5 1.5,-7.75; B6 3,-7.75; B7 4.5,-7.75
SOT23-5 = smd 0.55 x 1.2: 1 -0.95,-1.3; 2 0,-1.3; 3 0.95,-1.3; 4 0.95,1.3; 5 -0.95,1.3
SOT8 = smd 0.67 x 0.3: 1 -0.74,0.75; 2 -0.74,0.25; 3 -0.74,-0.25; 4 -0.74,-0.75; 5 0.74,-0.75; 6 0.74,-0.25; 7 0.74,0.25; 8 0.74,0.75
WSON-8-6X5-SKINNY_CENTERPAD = smd 0.85 x 0.5: 1 -2.775,1.905; 2 -2.775,0.635; 3 -2.775,-0.635; 4 -2.775,-1.905; 5 2.775,-1.905; 6 2.775,-0.635; 7 2.775,0.635; 8 2.775,1.905
WS2812-2020 = smd 0.7 x 0.7: DI -0.915,0.55; DO 0.915,-0.55; GND 0.915,0.55; VCC -0.915,-0.55
DFN-8 = smd 0.3 x 0.7: 1 -0.75,-0.99; 2 -0.25,-0.99; 3 0.25,-0.99; 4 0.75,-0.99; 5 0.75,0.99; 6 0.25,0.99; 7 -0.25,0.99; 8 -0.75,0.99 | smd 1.38 x 0.8: 9 0,0
SOT-23-6 = smd 0.55 x 1.35: 1 -0.95,-1.375; 2 0,-1.375; 3 0.95,-1.375; 4 0.95,1.375; 5 0,1.375; 6 -0.95,1.375
APS6404L-3SQR-ZR = smd 0.4 x 0.25: 1 -1.25,0.75; 2 -1.25,0.25; 3 -1.25,-0.25; 4 -1.25,-0.75; 5 1.25,-0.75; 6 1.25,-0.25; 7 1.25,0.25; 8 1.25,0.75 | smd 0.2 x 1.6: 9 0,0
CRYSTAL-SMD-2X2.5MM = smd 1.2 x 1.1: P1 0.846,0.69; P2 -0.854,0.69; P3 -0.854,-0.71; P4 0.846,-0.71

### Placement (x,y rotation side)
BOOT  16.51,9.53 90 top
C1  10.79,16.52 90 bottom
C2  15.88,16.52 90 bottom
C3  14.86,36.58 90 top
C4  17.66,38.73 0 top
C5  5.08,13.34 270 bottom
C6  3.81,19.68 0 bottom
C7  6.35,30.99 180 top
C8  13.34,36.2 0 top
C9  8.26,36.83 90 top
C10  6.99,24.77 0 bottom
C11  6.99,23.5 0 bottom
C12  6.35,32 180 top
C13  13.34,16.89 90 top
C14  16.51,27.94 0 top
C15  16.51,32.89 0 top
C16  12.78,26.34 270 top
C17  6.35,28.96 180 top
C18  11.24,36.96 90 top
C19  16.76,30.99 0 top
C20  7.62,25.15 90 top
C21  9.42,27.05 180 top
C22  6.35,27.81 180 top
C23  7.62,11.43 180 top
C24  15.88,16.89 90 top
C25  3.81,35.56 180 top
C26  11.43,19.05 180 top
D2  18.16,6.1 0 top
D3  7.62,12.7 0 top
D4  6.35,39.37 270 top
FB1  16.89,40.39 180 top
FD1  22.23,53.98 0 top
FD2  22.23,53.98 0 bottom
FD3  5.71,0.64 0 top
FD4  5.71,0.64 0 bottom
FRAME1  not placed on the board
H1  20.32,2.54 0 top
H2  2.54,2.54 0 top
H3  2.54,55.88 0 top
H4  20.32,55.88 0 top
I2C  1.27,8.89 270 bottom
J1  0,0 0 top
J2  3.81,17.78 90 top
J3  5.08,8.89 270 top
J4  11.43,6.35 0 top
J5  13.97,39.37 180 top
J6  12.06,11.18 0 bottom
L1  9.14,25.15 90 top
LOGO1  11.43,54.36 0 bottom
LOGO2  11.43,46.99 0 bottom
LOGO3  4.51,5.33 0 top
LOGO5  not placed on the board
LP  16.51,21.59 90 bottom
PWR  21.59,6.35 270 bottom
Q1  15.24,46.99 180 bottom
R1  3.81,40.63 270 top
R2  5.08,40.63 270 top
R3  13.34,7.87 270 top
R4  9.53,7.87 270 top
R5  3.17,7.63 90 bottom
R6  3.17,10.15 270 bottom
R7  9.53,16.52 90 bottom
R8  6.99,18.41 180 bottom
R9  13.33,37.47 180 top
R10  11.94,14.35 90 top
R11  10.92,14.35 90 top
R12  19.04,15.24 180 top
R13  15.25,25.4 0 top
R14  15.25,25.4 180 bottom
R15  20.95,6.1 180 top
R16  3.81,13.34 90 bottom
R17  2.54,13.34 90 bottom
R18  6.35,26.67 180 top
R19  4.45,38.1 0 top
R20  15.24,45.09 90 bottom
R21  15.88,19.05 90 top
R22  17.14,19.05 270 top
R23  11.81,25.4 180 bottom
RESET  20.95,9.53 270 top
SHLD  11.43,1.27 0 bottom
TP1  16.51,19.05 0 bottom
U1  11.43,31.75 180 top
U2  11.43,50.16 0 top
U3  13.34,16.51 90 bottom
U4  6.99,16.51 0 bottom
U5  11.43,21.59 0 bottom
U6  3.81,16.51 180 bottom
U7  6.35,36.2 90 top
U8  7.62,8.89 180 top
U9  14.61,13.97 270 top
U10  11.43,10.16 0 top
U11  11.43,21.59 270 top
U$1  [SDA0]  2.92,52.07 90 top
U$2  [SCL0]  2.92,49.53 90 top
U$3  [TX0]  19.94,49.53 90 top
U$4  [RX0]  19.94,47.24 90 top
U$5  [PICO0]  19.94,41.91 90 top
U$6  [POCI0]  19.94,44.7 90 top
U$7  [SCK0]  19.94,39.24 90 top
U$8  [#SDA_#0]  1.52,52.07 0 bottom
U$9  [#SCL_#0]  1.52,49.53 0 bottom
U$10  [#_TX#0]  21.34,49.53 0 bottom
U$11  [#_RX#0]  21.34,46.99 0 bottom
U$12  [#_POCI#0]  21.34,44.45 0 bottom
U$13  [#_PICO#0]  21.34,41.91 0 bottom
U$14  [#_SCK#0]  21.34,39.37 0 bottom
U$15  [#_GND#0]  11.43,39.62 90 bottom
U$16  [#_A0#0]  21.34,24.13 0 bottom
U$17  [#_3V3#0]  21.34,16.51 0 bottom
U$18  [##RST#_#0]  21.34,13.97 0 top
U$19  [#I2C#0]  1.27,10.29 90 bottom
U$20  [#_SWCLK#0]  13.97,39.62 90 bottom
U$21  [#_SWDIO#0]  8.89,39.62 90 bottom
U$22  [#_VB#0]  1.52,24.13 0 top
U$23  [#_VU#0]  1.52,29.21 0 top
U$24  [#_EN#0]  1.52,26.67 0 top
U$25  [#3V3_#0]  21.34,16.51 0 top
U$26  [#LP#0]  16.51,22.48 90 bottom
U$27  [#GND_#0]  21.34,21.59 0 top
U$28  [#11_#0]  21.34,34.29 0 top
U$29  [#26#A0_#0]  21.34,24.13 0 top
U$30  [#27#A1_#0]  21.34,26.67 0 top
U$31  [#28#A2_#0]  21.34,29.21 0 top
U$32  [BOOT0]  14.35,9.53 90 top
U$33  [RESET0]  18.8,9.53 90 top
U$34  [#VU_#0]  1.52,29.21 0 bottom
U$35  [#VB_#0]  1.52,24.13 0 bottom
U$36  [#EN_#0]  1.52,26.67 0 bottom
U$38  [#_A1#27#0]  21.34,26.67 0 bottom
U$39  [#_A2#28#0]  21.34,29.21 0 bottom
U$40  [#PWR#0]  20.95,6.35 0 bottom
U$41  [#SHLD#0]  11.43,2.92 0 bottom
U$42  [THING_PLUS0]  11.43,52.07 0 bottom
U$43  [RP23500]  11.43,50.16 0 bottom
U$44  [#_G#0]  21.34,21.59 0 bottom
U$45  [RP23500]  13.97,21.72 90 top
U$46  [#_16#0]  1.52,31.75 0 top
U$47  [#_17#0]  1.52,34.29 0 top
U$48  [#_18#0]  1.52,36.83 0 top
U$49  [CHG0]  5.08,12.7 0 top
U$50  [200]  2.92,41.91 90 top
U$51  [210]  2.92,44.45 90 top
U$52  [220]  2.92,46.99 90 top
U$53  [#22_#0]  1.52,46.99 0 bottom
U$54  [#21_#0]  1.52,44.45 0 bottom
U$55  [#20_#0]  1.52,41.91 0 bottom
U$56  [#19_#0]  1.52,39.37 0 bottom
U$57  [#18_#0]  1.52,36.83 0 bottom
U$58  [#17_#0]  1.52,34.29 0 bottom
U$59  [#16_#0]  1.52,31.75 0 bottom
U$60  [190]  2.92,39.37 90 top
U$61  [##RST#_#0]  21.59,13.72 90 bottom
U$62  [PWR0]  18.16,4.95 0 top
U$63  [STAT0]  7.37,39.37 90 top
U$64  [#5_#0]  21.34,31.75 0 top
U$65  [#12_#0]  21.34,36.83 0 top
U$66  [#_12#0]  21.34,36.83 0 bottom
U$67  [LED0]  19.94,52.07 90 top
U$68  [#_LED#0]  21.34,52.07 0 bottom
U$69  [#_5#0]  21.34,31.75 0 bottom
U$70  [#_11#0]  21.34,34.29 0 bottom
U$72  [#VA_#0]  21.34,19.05 0 top
U$73  [#_VA#0]  21.34,19.05 0 bottom
Y1  17.02,36.83 0 top

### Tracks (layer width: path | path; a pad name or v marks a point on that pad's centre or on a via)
1.1V  (via drill 0.3)
  Top 0.203: C7.1 7.21,31.35 U1.39 9.45,31.35 | C19.1 16.23,30.95 U1.6 14.21,30.95 v13.61,30.35 | C18.1 11.43,36.27 U1.23 11.43,34.27 11.21,34.05 v11.21,33.92 11.08,33.92 10.9,33.73 9.6,33.73 9.45,33.58 9.45,31.35 | 10.62,27.05 10.62,27.25 10.23,27.64 U1.50 10.23,29.14 9.45,29.92 9.45,31.35
  Top 0.508: C20.1 7.62,23.75 7.98,23.39 10.29,23.39 10.62,23.72 10.62,27.05
  Route15 0.203: v13.61,30.35 13.56,30.35 12.16,31.75 11.81,31.75 11.43,32.13 11.43,33.7 v11.21,33.92
  pour Top (isolate 0.127, no thermals): 10.11,23.95 10.11,24.89 7.42,24.89 7.42,24.41 8.28,24.41 8.28,23.95
3.3V  (via drill 0.3)
  Top 0.203: U1.30 8.63,35.95 C9.1 8.26,36.38 8.91,37.03 v8.97,37.03 | C12.1 7.1,31.75 U1.38 8.81,31.75 v8.94,31.88 | C21.1 9.83,27.14 U1.49 9.83,28.75 9.47,29.11 v9.47,29.16 | U1.1 15.25,28.95 16.01,28.19 C14.1 16.01,27.44 v15.49,26.92 14.61,26.04 13.51,26.04 12.78,26.76 C16.1 12.78,26.87 11.83,27.81 | U1.11 15.95,32.95 C15.1 16.54,32.36 17.76,32.36 v18.03,32.64 | C8.1 12.63,35.99 U1.20 12.63,34.65 v12.32,34.34 | U1.53 11.43,27.96 11.58,27.81 11.83,27.81 | U1.54 11.83,27.81 | v5.21,26.04 R18.2 | R13.2 v17.02,25.4 | v5.8,29.68 6.25,29.68 6.85,29.08 C17.1 U1.45 | R12.2 18.16,15.62 v17.78,15.62 | D2.A 17.28,4.58 v17.27,4.57 | C26.1 11.93,19.68 12.18,19.93 U11.8 12.5,20.34 12.7,20.14 v12.83,20.14
  Bottom 0.203: Q1.2 15.74,48.76 v15.88,48.9 | R8.2 6.99,18.92 v6.99,22.48 7.49,22.98 C11.1 | C11.1 U5.8 | C11.1 C10.1 | R23.2 12.31,26.54 14.5,28.73 | LP.2 16.51,22.87 17.02,23.38 v17.02,25.4
  Bottom 0.508: v15.49,26.92 15.49,27.74 14.5,28.73 v14.02,29.21 | v8.97,37.03 8.97,37.05 9.38,37.47 10.03,37.47 12.32,35.18 | 12.32,35.18 v12.32,34.34 | 12.32,35.18 16.89,39.75 v16.89,40.01 v16.89,40.77
  other vias: 15.16,16.26 14.63,16.26
  pour Route15 (isolate 0.178, rank 2): 0,0 22.86,0 22.86,53.59 0,53.59
  pour Top (isolate 0.203, no thermals): 16.64,40.89 16.64,39.88 16.76,39.75 17.14,39.75 17.27,39.88 18.03,39.88 18.03,40.89 17.27,40.89 17.14,41.02 16.76,41.02
  pour Bottom (isolate 0.203, no thermals): 14.55,16.43 14.15,16.03 14.15,15.57 14.33,15.39 15.67,15.39 16.08,15.8 16.08,16.18 15.82,16.43
3.3V_SW  (via drill 0.3)
  Top 0.203: U7.VCC 6.16,34.54 5.46,34.54 v4.95,35.05 4.45,35.56 C25.1
  Top 0.508: J3.2 5.66,9.39 6.22,9.95 v6.22,10.67 v6.22,11.18 | v14.86,14.22 v14.86,14.73 15.05,14.92 U9.5 15.9,16.36 C24.1
  Route15 0.203: v4.19,30.48 4.19,23.75 6.99,20.95 6.99,19.94 10.16,16.76 v10.16,13.97
  Bottom 0.203: v6.22,10.67 4.45,8.89 I2C.2 | v4.95,35.05 5.59,34.42 5.59,32.13 5.33,31.88 4.83,31.88 4.19,31.24 v4.19,30.48
  Bottom 0.305: 8.64,11.18 8.64,8 8.76,7.87 8.76,6.6 9.02,6.35 10.71,6.35 11.16,6.81 J6.4
  Bottom 0.508: v6.22,10.67 v6.22,11.18 8.64,11.18 10.16,12.7 v10.16,13.97 10.41,14.22 v14.86,14.22 v14.86,14.73
!BATT_ALERT!  (via drill 0.3)
  Top 0.203: U1.19 13.03,34.09 v12.9,33.96 | v6.17,8.08 6.82,8.08 6.87,8.03 U8.5
  Route15 0.203: v9.27,10.29 8.38,10.29 v6.17,8.08
  Bottom 0.203: v12.9,33.96 13.74,34.8 14.22,34.8 15.88,33.15 15.88,30.1 17.02,28.96 17.02,27.69 18.29,26.42 18.29,13.08 17.02,11.81 14.1,11.81 13.84,12.06 12.06,12.06 10.29,10.29 v9.27,10.29
!BOOT!  (via drill 0.3)
  Top 0.203: BOOT.4 BOOT.3 15.71,11.6 14.86,12.45 v14.86,12.95
  Bottom 0.203: v14.86,12.95 15.24,12.95 16.76,14.48 16.76,17.53 16.51,17.78 TP1.1 15.24,20.32 15.24,23.5 15.75,24 R14.2
!RESET!  (via drill 0.3)
  Top 0.203: U1.26 10.23,34.6 v10.59,34.24 | v17.78,17.78 19.54,16.02 R12.1 20.32,15.24 J1.28 21.59,11.74 RESET.4 RESET.3
  Bottom 0.203: v10.59,34.24 10.59,33.35 10.92,33.02 13.99,33.02 14.73,32.28 14.73,29.97 16,28.7 16,27.43 17.53,25.91 17.53,20.7 17.27,20.45 17.27,19.94 17.78,19.43 v17.78,17.78
BAT_SW  (via drill 0.3)
  Route15 0.203: v6.35,20.32 3.43,23.24 v3.43,30.48
  Bottom 0.203: U4.8 6.25,17.66 6.49,17.91 R8.1 6.49,18.91 6.35,19.05 v6.35,20.32 | v3.43,30.48 3.43,30.99 4.57,32.13 4.57,33.66 4.06,34.16 4.06,37.59 4.57,38.1 4.57,41.15 5.84,42.42 5.84,49.15 6.1,49.4 6.82,49.4 8.14,48.09 Q1.1
EN  (via drill 0.3)
  Top 0.203: v7.62,21.34 5.33,21.34 3.81,22.86 3.81,24.13 J1.11
  Bottom 0.203: U3.3 11.65,17.46 11.46,17.65 10.16,17.65 R7.2 8.26,18.29 8.26,18.92 7.62,19.56 v7.62,21.34
GND  (via drill 0.3)
  Top 0.203: U2.A7 4.91,43.94 5.46,43.94 5.97,44.45 v7.87,44.45 | U8.6 7.37,8.64 U8.9 | U8.9 7.87,8.89 8.37,9.39 U8.1 | C23.2 7.12,10.57 6.89,10.34 6.89,9.9 U8.4 6.87,9.39 7.37,8.89 U8.9 | J4.GND2 14.92,5.74 14.92,4.45 v14.95,4.42 | J4.GND 7.94,5.74 7.94,4.45 v7.91,4.42 | U1.EPAD v10.79,32.38 | v5.08,31.37 5.59,31.88 5.72,31.88 C12.2 | 12.47,13.97 12.47,12.62 12.63,12.47 13.21,12.47 | U9.2 12.47,13.97 | v11.43,24.13 11.43,23.75 10.68,23 U11.4 10.68,22.36 10.41,22.1 10.41,21.84 10.67,21.59 U11.9 12.45,21.59 12.7,21.34 v12.7,20.95 | C15.2 17.52,33.4 v17.78,33.4 | C16.2 13.22,25.4 v13.97,25.4 | v14.99,18.16 13.66,18.16 13.34,17.84 C13.2 12.88,17.39 12.47,16.98 12.47,13.97
  Top 0.305: v4.99,11.41 5.39,11.81 6.74,11.81 C23.2 7.62,11.93 7.62,12.19 | U10.2 v11.43,10.41
  Top 0.508: C8.2 v14.35,36.2 14.46,36.08 C3.1
  Route2 0.203: 9.36,29.76 8.93,29.34 | 9.4,31.37 8.51,31.37
  Bottom 0.203: 15.98,14.33 16.4,14.75 16.4,16.49 C2.2 15.75,16.89 14.2,16.89 v14.05,16.74 | v10.79,31.11 10.62,31.11 8.55,29.04 5.04,29.04 v4.95,28.96 | 9.27,31.37 8.38,31.37
  Bottom 0.508: U3.2 11.56,16.51 11.05,17.02 C1.2
  other vias: 12.06,32.38 12.06,31.11 11.28,26.21 9.63,36.78 5.08,42.55 18.29,31.11 12.04,37.52 8.13,26.92 7.62,26.42 6.73,25.65 6.99,53.34 8.26,53.34 9.53,53.34 10.79,53.34 12.06,53.34 13.34,53.34 14.61,53.34 15.88,53.34 2.54,53.34 20.32,53.34 2.54,48.26 18.16,42.8 17.78,14.86 5.08,30.73 4.95,27.94 4.95,37.08 17.78,27.81 6.11,8.89 3.81,18.92 9.57,9.5 14.35,8.76 14.22,12.45 5.97,13.59 10.41,18.16 2.54,30.48 16.26,45.72 18.8,39.37 16.26,8.89 18.41,0.64 22.23,4.45 4.45,0.64 0.64,4.45 8.26,0.64 14.61,0.64 20.32,10.16 16.51,48.26 20.32,50.8 7.87,46.35 14.35,46.74 1.91,18.92 3.3,11.43 18.8,35.31 8.1,35.08 5.71,24.13 6.99,17.75 7.75,22.48
  pour Top (isolate 0.178, rank 2): 0,0 22.86,0 22.86,53.59 0,53.59
  pour Bottom (isolate 0.178, rank 2): 22.86,0 0,0 0,53.59 22.86,53.59
  pour Route2 (isolate 0.178, rank 2): 0,0 22.86,0 22.86,53.59 0,53.59
  pour Top (isolate 0.127, no thermals): 9.07,28.55 9.07,26.82 8.76,26.82 7.82,25.88 7.82,25.4 7.39,25.4 7.39,27.05 7.85,27.51 8.86,27.51 8.99,27.64 8.99,28.55
GPIO5  (via drill 0.3)
  Top 0.203: U1.8 15.37,31.75 15.62,32 17.91,32 18.29,32 v18.8,32.51
  Route15 0.203: v18.8,32.51 20.57,32.51 21.34,31.75 J1.21
GPIO11  (via drill 0.3)
  Top 0.203: U1.15 16.23,34.55 16.3,34.62 16.94,34.62 v17.14,34.42
  Route15 0.203: J1.20 17.27,34.29 v17.14,34.42
GPIO12  (via drill 0.3)
  Top 0.203: v17.78,34.8 17.39,35.19 U1.16
  Route15 0.203: J1.19 19.56,34.8 v17.78,34.8
GPIO16  (via drill 0.3)
  Top 0.203: U1.27 9.83,35.89 v9.63,36.09
  Route15 0.203: v9.63,36.09 9.63,35.46 9.5,35.33 9.5,34.14 9.17,33.81 2.56,33.81 2.03,33.27 2.03,32.51 J1.9
GPIO17  (via drill 0.3)
  Top 0.203: U1.28 9.43,34.7 9.04,34.31 v8.89,34.31
  Route15 0.203: v8.89,34.31 8.76,34.19 1.37,34.19 J1.8
GPIO18  (via drill 0.3)
  Top 0.203: U1.29 9.03,36.28 v8.97,36.35
  Route15 0.203: J1.7 3.56,34.54 8.38,34.54 8.97,35.13 v8.97,36.35
GPIO19
  Top 0.203: U1.31 7.1,34.55 6.72,34.17 3.3,34.17 2.54,34.92 2.54,38.1 J1.6
GPIO20  (via drill 0.3)
  Top 0.203: v2.54,32.77 2.54,33.53 2.78,33.77 6.85,33.77 7.23,34.15 U1.32
  Bottom 0.203: v2.54,32.77 2.54,40.64 J1.5
GPIO21  (via drill 0.3)
  Top 0.203: v3.05,33.25 3.17,33.37 6.98,33.37 7.36,33.75 U1.33
  Bottom 0.203: v3.05,33.25 2.92,33.38 2.92,42.8 J1.4
GPIO22  (via drill 0.3)
  Top 0.203: U1.34 7.49,33.35 7.1,32.97 3.76,32.97 v3.56,32.77
  Bottom 0.203: v3.56,32.77 3.56,33.53 3.3,33.78 3.3,44.96 J1.3
GPIO26/A0  (via drill 0.3)
  Top 0.203: U1.40 8.78,30.95 v8.89,30.84
  Route15 0.203: v8.89,30.84 8.38,30.33 8.38,29.95 8.74,29.59 9.14,29.59 9.25,29.69 9.7,29.69 11.46,27.94 16.13,27.94 17.4,26.67 19.05,26.67 J1.24
GPIO27/A1  (via drill 0.3)
  Top 0.203: U1.41 8.44,30.55 8.84,30.15 v8.94,30.15
  Route15 0.203: v8.94,30.15 9.73,30.15 11.56,28.32 19.94,28.32 J1.23
GPIO28/A2  (via drill 0.3)
  Top 0.203: U1.42 7.18,30.15 v7.07,30.26
  Route15 0.203: v7.07,30.26 8.18,31.37 9.27,31.37 9.53,31.11 9.53,30.84 11.66,28.7 19.81,28.7 20.32,29.21 J1.22
LED_IN  (via drill 0.3)
  Top 0.203: U7.DI 4.95,36.13 v4.95,36.2 | U1.18 13.43,33.76 v13.56,33.64
  Route15 0.203: v13.56,33.64 13.35,33.43 12.41,33.43 11.81,34.04 11.81,36.32 10.29,37.85 6.6,37.85 v4.95,36.2
LED_OUT  (via drill 0.3)
  Top 0.203: U7.DO 6.73,36.94 6.73,36.58 v6.48,36.32
  Bottom 0.203: v6.48,36.32 6.48,40.77 7.37,41.66 7.37,46.61 8.25,47.49 17.01,47.49 19.05,49.53 19.05,50.8 20.32,52.07 J1.13
N$1
  Top 0.508: U2.C2 16.77,45.22 15.93,44.38 U2.B7 15.93,40.45 FB1.2
N$2
  Top 0.203: U2.A6 4.17,45.22 3.43,44.47 3.43,41.51 R1.1
N$3
  Top 0.203: R2.1 6.1,42.15 6.1,43.56 6.35,43.81 9.04,43.81 9.93,42.92 U2.B3
N$4
  Top 0.203: R19.2 5.96,38.1 D4.C
N$5
  Top 0.203: J4.B5 13.18,7.21 R3.2
N$6
  Top 0.203: J4.A5 10.18,6.71 R4.2
N$7
  Top 0.233: R11.1 10.9,13.83 10.9,12.27 10.48,11.86 U10.6 | J4.A7 11.68,5.46 11.43,5.21 10.92,5.21 10.68,5.45 J4.B7 10.68,6.74 11.16,7.22 11.16,7.72 10.48,8.4 U10.1
  Top 0.508: U10.1 U10.6
N$8
  Top 0.233: R10.1 11.96,13.83 11.96,12.27 12.38,11.86 U10.4 | J4.A6 11.18,6.61 11.68,7.11 | J4.B6 12.18,6.62 11.68,7.11 | 11.68,7.11 11.68,7.71 12.38,8.4 U10.3
  Top 0.508: U10.3 U10.4
N$9
  Bottom 0.203: I2C.3 2.26,7.85 2.54,8.13 R5.2
N$10
  Bottom 0.203: I2C.1 2.26,9.93 2.54,9.65 R6.2
N$11  (via drill 0.3)
  Top 0.203: v16.13,20.32 15.88,20.07 R21.2
  Bottom 0.203: LP.1 16.13,20.69 v16.13,20.32
N$13
  Top 0.203: U1.21 12.23,36.49 12.57,36.83 14.61,36.83 C3.2 15.44,36.5 15.78,36.5 Y1.P3
N$14
  Top 0.203: Y1.P1 17.36,38.03 17.36,38.54 C4.1 15.86,38.73 14.84,37.72 14.08,37.72 R9.1
N$15
  Top 0.203: U1.22 11.83,36.57 12.72,37.47 R9.2
N$18
  Top 0.203: R15.2 D2.C
N$19  (via drill 0.3)
  Top 0.203: R15.1 21.59,5.96 v21.59,5.08
  Bottom 0.203: PWR.2 v21.59,5.08
N$20
  Bottom 0.203: R16.2 2.86,14.79 U6.5
N$21  (via drill 0.3)
  Top 0.203: v3.3,12.19 3.81,12.7 D3.A
  Bottom 0.203: R17.1 3.18,12.19 v3.3,12.19
N$22  (via drill 0.3)
  Top 0.203: D3.C 8.5,13.46 8.12,13.84 8.12,14.86 7.1,15.88 5.21,15.88 3.3,17.78 v1.91,17.78
  Bottom 0.203: U6.1 1.94,17.81 v1.91,17.78
N$23
  pour Top (isolate 0.127, no thermals): 8.94,25.7 9.78,25.7 9.78,26.29 9.47,26.59 9.47,28.32 9.4,28.32 9.4,26.67 8.94,26.21
PERIPH_POW  (via drill 0.3)
  Top 0.203: U9.3 14.19,13.02 14.7,13.53 15.05,13.53 15.49,13.97 16.51,13.97 17.14,14.61 R22.2 16.51,18.55 | 16.51,18.55 R21.1 | 16.51,18.55 16.51,19.94 16.76,20.19 v17.78,20.19 | U1.17 13.83,34.43 v13.97,34.29
  Bottom 0.203: v17.78,20.19 17.91,20.32 17.91,26.16 16.45,27.62 16.45,28.89 15.24,30.1 15.24,33.02 v13.97,34.29
PICO  (via drill 0.3)
  Top 0.203: J1.17 19.81,40.13 19.81,31.75 18.48,30.42 v17.91,30.42 15.88,30.42 15.76,30.55 U1.5
  Bottom 0.203: J6.3 10.41,7.49 13.59,10.67 17.78,10.67 19.43,12.32 19.43,28.32 17.91,29.84 v17.91,30.42
POCI  (via drill 0.3)
  Top 0.203: J1.16 19.3,42.16 19.3,32.13 v18.92,31.75 18.8,31.62 15.75,31.62 15.47,31.35 U1.7
  Bottom 0.203: J6.7 14.81,8.46 16.26,9.91 18.29,9.91 20.19,11.81 20.19,29.08 18.92,30.35 v18.92,31.75
PSRAM_!CS!  (via drill 0.3)
  Top 0.203: U1.12 14.43,33.35 v13.59,32.51 | U11.1 12.18,23.51 v12.06,23.62
  Bottom 0.203: v13.59,32.51 14.22,31.88 14.22,30.18 13.51,29.46 13.51,28.5 11.81,26.8 11.81,25.9 R23.1 12.06,24.65 v12.06,23.62
QSPI_!CS!  (via drill 0.3)
  Top 0.203: U1.60 14.23,27.55 v14.73,27.05 | R14.1 14.99,25.16 v14.99,24.64
  Bottom 0.203: U5.1 14.33,23.5 14.99,24.15 v14.99,24.64 14.99,25.16 R14.1 14.73,25.42 v14.73,27.05
QSPI_CLK  (via drill 0.3)
  Top 0.203: U1.56 12.63,28.98 12.19,29.41 v12.19,29.59 | U11.6 11.18,20.57 10.92,20.83 10.03,20.83 v9.53,21.34
  Bottom 0.203: v12.19,29.59 12.19,28.45 10.05,26.31 10.05,21.86 v9.53,21.34 9.4,21.21 9.14,21.21 8.89,20.95 U5.6
QSPI_D0  (via drill 0.3)
  Top 0.203: v12.88,29.46 13.03,29.31 U1.57 | U11.5 9.54,20.34 v9.53,20.32
  Bottom 0.203: v12.88,29.46 12.88,28.63 10.56,26.31 10.56,21.36 v9.53,20.32 8.89,19.68 U5.5
QSPI_D1  (via drill 0.3)
  Top 0.203: U1.59 13.83,27.32 14.22,26.92 v14.22,26.54 | U11.2 11.68,22.61 11.94,22.35 12.95,22.35 v13.46,22.86
  Bottom 0.203: v14.22,26.54 13.46,25.78 v13.46,22.86 14.1,22.23 U5.2
QSPI_D2  (via drill 0.3)
  Top 0.203: U11.3 11.18,22.48 11.68,21.97 12.83,21.97 v12.95,21.84 | U1.58 13.43,26.87 v13.55,26.75
  Bottom 0.203: U5.3 14.08,20.95 13.57,21.46 13.34,21.46 v12.95,21.84 12.95,26.16 v13.55,26.75
QSPI_D3  (via drill 0.3)
  Top 0.203: U1.55 12.23,28.77 11.51,29.49 v11.51,29.59 | U11.7 11.68,20.7 11.18,21.21 10.54,21.21 v9.53,22.23
  Bottom 0.203: v11.51,29.59 11.51,28.27 9.54,26.31 9.54,22.24 v9.53,22.23 U5.7
RX  (via drill 0.3)
  Top 0.203: U1.3 15.5,29.75 15.88,29.37 18.83,29.37 v20.32,30.86
  Bottom 0.203: v20.32,30.86 20.32,45.72 J1.15
SCK  (via drill 0.3)
  Top 0.203: U1.4 15.63,30.15 15.88,29.9 v18.59,29.9 20.32,31.62 20.32,38.1 J1.18
  Bottom 0.203: J6.5 12.62,7.92 14.99,10.29 18.03,10.29 19.81,12.06 19.81,28.68 v18.59,29.9
SCL  (via drill 0.3)
  Top 0.203: U1.10 14.36,32.55 v13.59,31.77 | U8.7 7.87,7.57 7.57,7.26 6.22,7.26 6.1,7.39 J3.4 v5.08,6.6 | v2.29,10.67 2.29,7.24 v3.17,6.35
  Route15 0.203: J1.2 2.54,49.53 4.45,47.62 7.87,47.62 15.49,40.01 15.49,35.53 14.81,34.85 14.81,32.69 13.89,31.77 v13.59,31.77
  Bottom 0.203: v5.08,6.6 4.33,6.6 3.81,7.13 R5.1 v3.17,6.35 | v13.59,31.77 13.49,31.77 12.19,30.48 10.92,30.48 10.54,30.1 10.54,29.21 9.91,28.57 6.35,28.57 3.81,26.04 3.81,22.23 0.76,19.18 0.76,12.19 v2.29,10.67
SD_!CS!  (via drill 0.3)
  Top 0.203: v17.02,33.66 16.89,33.53 16.26,33.53 16.03,33.75 U1.13
  Bottom 0.203: v17.02,33.66 17.02,30.23 19.05,28.19 19.05,12.57 17.53,11.05 12.88,11.05 9.31,7.48 J6.2
SD_DET  (via drill 0.3)
  Top 0.203: v13.59,11.56 v13.59,9.91 | v16.51,34.12 16.48,34.15 U1.14
  Bottom 0.203: J6.9 11.87,8.18 v13.59,9.91 | v13.59,11.56 13.72,11.43 17.27,11.43 18.67,12.83 18.67,27.94 16.51,30.1 v16.51,34.12
SDA  (via drill 0.3)
  Top 0.203: U1.9 14.44,32.15 14.18,31.9 14.18,31.43 13.82,31.06 v13.59,31.06 | U8.8 8.37,7.56 7.67,6.86 6.1,6.86 5.33,6.1 4.83,6.1 4.06,6.86 4.06,7.75 4.71,8.39 J3.3 4.69,8.39 3.94,9.14 v3.94,9.53
  Route15 0.203: J1.1 5.08,48.26 8,48.26 15.94,40.32 15.94,35.24 15.3,34.61 15.3,32.45 13.92,31.06 v13.59,31.06
  Bottom 0.203: v3.94,9.53 3.94,9.89 R6.1 1.27,12.56 1.27,19.05 4.32,22.1 4.32,25.91 6.6,28.19 10.16,28.19 10.99,29.02 10.99,29.91 11.18,30.1 12.62,30.1 v13.59,31.06
SHLD
  Bottom 0.203: J4.SHLD3 7.13,1.27 SHLD.2
  pour Route2 (isolate 0.203): 7.11,5.59 7.11,1.14 15.75,1.14 15.75,5.59
SWCLK
  Top 0.203: U1.24 11.03,35.71 10.67,36.07 10.67,37.85 10.92,38.1 12.7,38.1 J5.1
SWDIO
  Top 0.203: J5.3 10.25,38.01 10.25,36 10.63,35.62 U1.25
TX  (via drill 0.3)
  Top 0.203: U1.2 15.37,29.35 15.76,28.97 19.19,28.97 v20.32,30.1
  Bottom 0.203: v20.32,30.1 19.81,30.61 19.81,47.75 J1.14
USB_D_N
  Top 0.233: U1.51 10.63,27.75 11.81,26.57 11.81,25.27 13.08,24 13.72,24 14.48,23.24 14.48,20.07 11.25,16.84 11.25,15.18 R11.2
USB_D_P
  Top 0.233: U1.52 11.03,27.86 12.17,26.72 12.17,25.42 13.23,24.36 13.87,24.36 14.84,23.39 14.84,19.92 11.61,16.69 11.61,15.18 R10.2
V_BATT  (via drill 0.3)
  Top 0.203: U8.3 7.37,10.16 7.62,10.41 | 7.62,10.41 7.87,10.16 U8.2 | 7.62,10.41 8.12,10.91 C23.1 8.76,11.43 9.26,11.94 9.26,13.34 8.64,13.97 v8.64,15.75
  Top 0.305: v8.64,15.75 8.64,16.51 8.37,16.78 J2.1
  Top 0.508: v4.76,18.92 4.76,17.59 5.57,16.78 J2.1
  Route15 0.508: J1.12 1.27,22.41 v4.76,18.92 7.93,15.75 v8.64,15.75
  Bottom 0.305: U4.3 8.38,16.26 8.64,16 v8.64,15.75
  Bottom 0.508: U6.3 v4.76,18.92 4.76,19.23 C6.1
V_USB  (via drill 0.3)
  Top 0.305: U10.5 v11.43,12.7
  Route15 0.508: J1.10 2.54,27.94 2.54,22.86 6.35,19.05 6.73,19.05 9.4,16.38 9.4,14.73 | 9.4,14.73 v5.84,14.73 | 9.4,14.73 9.4,13.46 10.16,12.7 v11.43,12.7 11.43,11.43 10.41,10.41 10.41,9.14 9.4,8.13 v9.4,4.95 9.65,4.7 v10.54,4.7 v12.32,4.7 13.21,4.7 v13.46,4.95
  Bottom 0.203: R17.2 2.16,14.22 2.16,15.88 2.54,16.26 4.06,16.26 4.76,15.56 U6.4
  Bottom 0.305: U6.4 4.76,15.46 5.56,16.26 U4.6
  Bottom 0.508: U6.4 4.76,14.15 C5.1 5.84,14.6 v5.84,14.73
  pour Top (isolate 0.203, no thermals): 8.76,6.35 8.76,5.21 9.53,4.45 13.34,4.45 14.1,5.21 14.1,6.35
VDDA  (via drill 0.3)
  Top 0.203: R18.1 C22.1 7.03,27.64 v7.75,27.64 8.33,27.64 8.63,27.93 U1.46 8.63,28.75 8.66,28.78 8.66,29.12 8.43,29.35 U1.44
  Route15 0.203: v7.75,27.64 8.94,27.64 9.02,27.56 15.88,27.56 17.65,25.78 17.65,22.99 J1.26
VIN  (via drill 0.3)
  Top 0.508: U9.1 13.3,15.4 v13.08,15.62 13.34,15.88 C13.1
  Bottom 0.305: U4.7 U4.2 8.78,16.76 R7.1
  Bottom 0.508: R7.1 C1.1 11.25,15.56 U3.1 13.02,15.56 v13.08,15.62
WL_CLK  (via drill 0.3)
  Top 0.203: U2.A3 6.04,49.72 6.35,49.4 v6.35,48.9 | v6.35,30.23 6.83,29.75 U1.43
  Bottom 0.203: v6.35,48.9 6.86,48.39 6.86,41.91 5.97,41.02 5.97,35.94 6.35,35.56 6.35,34.42 6.99,33.78 6.99,31.62 6.35,30.99 v6.35,30.23
WL_CS  (via drill 0.3)
  Top 0.203: U2.B2 8.43,41.83 v7.49,40.89 | U1.37 8.48,32.15 8.91,32.59 v8.94,32.59
  Bottom 0.203: v8.94,32.59 8.91,32.59 6.99,34.52 6.99,40.39 v7.49,40.89
WL_D  (via drill 0.3)
  Top 0.203: U1.36 5.25,32.55 v5.08,32.38 | R1.2 R2.2 v5.08,39.37 | v6.35,46.61 6.24,46.72 U2.A5
  Bottom 0.203: v5.08,32.38 5.08,33.78 4.45,34.42 4.45,37.34 5.08,37.97 v5.08,39.37 5.08,40.89 6.35,42.16 v6.35,46.61
WL_GPIO0
  Top 0.203: D4.A 6.93,40.83 U2.B1
WL_GPIO2  (via drill 0.3)
  Top 0.203: U2.C3 16.28,46.72 v16.26,46.74
  Bottom 0.203: R20.2 Q1.3 16.05,46.94 v16.26,46.74
WL_ON  (via drill 0.3)
  Top 0.203: U2.B6 U2.B5 12.93,41 v12.83,40.89 | U1.35 8.57,32.95 8.91,33.3 v8.94,33.3
  Bottom 0.203: v12.83,40.89 8.51,40.89 7.59,39.98 7.59,34.65 v8.94,33.3

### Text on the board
Bottom: v10
tDocu: 4-layer / JLC7628 Stackup / Material: TG135-140 / 1oz outer layers / 0.5oz inner layers / Board thickness: 1.6mm / Soldermask: Red / Silkscreen: White / Surface Finish: Lead-Free HASL | Dryw Wade | Based on design by: Nathan Seidle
